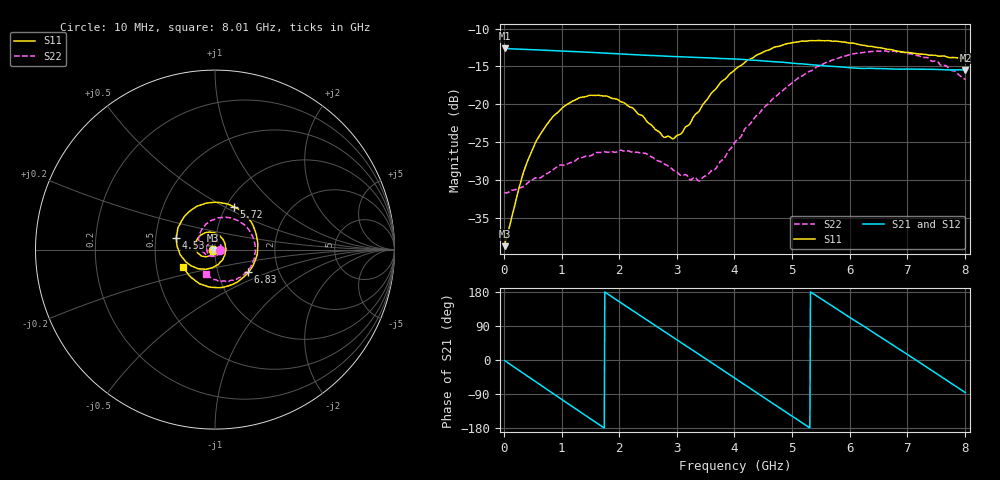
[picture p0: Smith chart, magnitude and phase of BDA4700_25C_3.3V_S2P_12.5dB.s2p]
!Agilent Technologies,E5071B,MY42404982,A.09.10
!Date: Mon Oct 20 18:08:16 2025
!Data & Calibration Information:
!Freq	S11:SOLT2(ON)	S21:SOLT2(ON)	S12:SOLT2(ON)	S22:SOLT2(ON)
# Hz S RI R 50
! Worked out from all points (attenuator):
!   801 points, 10 MHz to 8.01 GHz, reference 50 ohm
!   highest |S21| = -12.60 dB at 10 MHz (marker M1); lowest = -15.5 dB at 8.01 GHz (marker M2)
!   lowest |S11| = -38.7 dB at 10 MHz (marker M3), VSWR 1.02, Z = 48.9 - j0.164 ohm
!   |S11| at or under -10 dB: start of sweep to end of sweep
!   |S22| runs from -31.7 to -12.9 dB; largest |S21 - S12| = 0.0027
!   S11 on the Smith chart (normalised r, x): 10 MHz: 0.98, -0.00; 4.53 GHz: 0.64, +0.08; 5.72 GHz: 1.09, +0.56; 6.83 GHz: 1.40, -0.37; 8.01 GHz: 0.69, -0.14
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1e7  -0.0115 -0.00168  0.2343 -0.00512  0.2343 -0.00534  0.0263 -0.000943
3.3e8  -0.0224 -0.0268  0.1898 -0.1315  0.1896 -0.1316  0.0228 -0.0172
5.6e8  -0.0422 -0.0389  0.1196 -0.1951  0.1194 -0.1952  0.0144 -0.0294
8.7e8  -0.0771 -0.0345  -0.00184 -0.2263  -0.00175 -0.2263  -0.00912 -0.0365
1.35e9  -0.1098 0.0205  -0.1693 -0.1435  -0.1693 -0.1435  -0.0421 -0.0143
1.65e9  -0.0945 0.065  -0.2158 -0.0367  -0.216 -0.0367  -0.0465 0.0125
1.94e9  -0.0555 0.0937  -0.2032 0.0734  -0.2032 0.0735  -0.0322 0.0361
2.33e9  0.0118 0.0854  -0.1083 0.1823  -0.1084 0.1823  0.00041 0.0482
2.68e9  0.0544 0.0383  0.0164 0.2086  0.0161 0.2085  0.0274 0.0322
2.95e9  0.0576 -0.016  0.1083 0.1764  0.1081 0.176  0.0349 0.0105
3.39e9  0.00241 -0.0907  0.1973 0.0504  0.1978 0.0504  0.0182 -0.0253
3.67e9  -0.0634 -0.1085  0.1958 -0.0482  0.1958 -0.0487  -0.00798 -0.0367
4.01e9  -0.1502 -0.0779  0.1328 -0.1487  0.133 -0.1483  -0.0476 -0.0296
4.53e9  -0.2157 0.0629  -0.0363 -0.1899  -0.036 -0.1903  -0.0902 0.0345
4.92e9  -0.1688 0.1866  -0.1447 -0.1207  -0.1441 -0.1216  -0.0772 0.1064
5.35e9  -0.0336 0.2607  -0.1823 0.0102  -0.1825 0.00911  -0.00465 0.1678
5.72e9  0.1046 0.2391  -0.1368 0.1138  -0.1368 0.1139  0.0893 0.1758
6.22e9  0.2267 0.096  -0.00525 0.1725  -0.00278 0.173  0.1984 0.0942
6.68e9  0.217 -0.0781  0.1184 0.1239  0.1189 0.124  0.2209 -0.0312
6.83e9  0.1853 -0.1268  0.1455 0.0897  0.1461 0.0889  0.2094 -0.0716
7.43e9  -0.0156 -0.2104  0.1506 -0.0799  0.1505 -0.0802  0.0868 -0.1721
8.01e9  -0.1761 -0.0964  0.0107 -0.1682  0.0114 -0.1683  -0.0504 -0.1366
